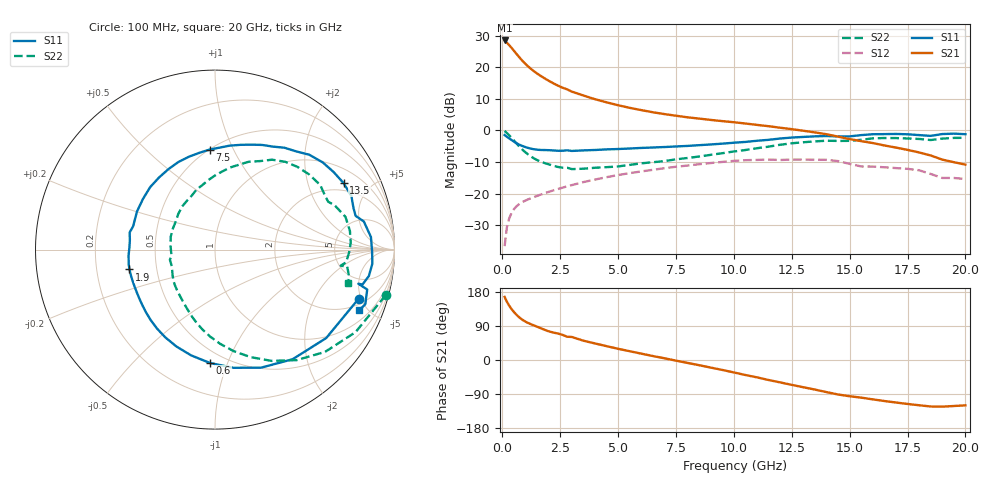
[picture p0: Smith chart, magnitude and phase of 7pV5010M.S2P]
! Infineon Technologies  Discrete & RF Semiconductors
! bfp620
! VCE = 0.50 V,  IC =  10 mA
! Common Emitter S-Parameters:  Sep 2002
# GHz  S  MA  R  50
!  f  S11  S21  S12  S22
! GHz  MAG  ANG  MAG  ANG  MAG  ANG  MAG  ANG
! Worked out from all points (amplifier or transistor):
!   59 points, 100 MHz to 20 GHz, reference 50 ohm
!   highest |S21| = 28.5 dB at 100 MHz (marker M1)
!   |S21| within 3 dB of that: start of sweep to 474.6 MHz
!   unconditionally stable (mu >= 1): 3.938 GHz to 10.17 GHz; 17.11 GHz to end of sweep
!   at 1 GHz: K = 0.51, MSG = 21.6 dB, |S12| = -22.2 dB
!   at 5.5 GHz: K = 1.05, MAG = 8.9 dB, |S12| = -13.5 dB
!   at 20 GHz: K = 1.68, MAG = -2.5 dB, |S12| = -15.4 dB
!   S11 on the Smith chart (normalised r, x): 100 MHz: 2.49, -4.79; 600 MHz: 0.41, -0.87; 1.9 GHz: 0.35, -0.10; 7.5 GHz: 0.50, +0.81; 13.5 GHz: 1.60, +3.40; 20 GHz: 1.58, -4.44
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0.1  0.8462 -18.8  26.47 166.4  0.0148 79.7  0.9837 -15.0
0.2  0.7917 -38.5  24.32 153.5  0.0297 69.7  0.9083 -30.4
0.3  0.7484 -54.7  22.26 143.1  0.0409 63.1  0.8372 -42.9
0.4  0.7062 -68.6  20.22 134.4  0.0497 57.7  0.7652 -53.6
0.5  0.6667 -81.1  18.26 126.8  0.0567 53.2  0.6952 -63.1
0.6  0.6324 -92.5  16.46 120.1  0.0625 49.6  0.6309 -71.7
0.7  0.6042 -102.7  14.86 114.3  0.0672 46.8  0.5744 -79.7
0.8  0.5811 -111.7  13.47 109.2  0.0713 44.6  0.5261 -86.8
1  0.5456 -126.4  11.27 101.2  0.0779 41.8  0.4508 -98.9
1.2  0.5194 -137.8  9.673 95.4  0.0837 40.2  0.3963 -108.6
1.4  0.5017 -147.3  8.47 90.4  0.0893 39.2  0.3563 -117.2
1.9  0.4891 -166.9  6.419 78.0  0.1038 37.1  0.2992 -138.1
2.6  0.4773 173.5  4.75 66.4  0.1245 34.2  0.2575 -160.6
2.8  0.4851 168.7  4.459 61.4  0.1308 33.0  0.2575 -167.4
3.5  0.4837 154.0  3.57 51.0  0.1525 28.7  0.2482 175.9
5  0.5087 127.7  2.504 29.6  0.1973 17.5  0.2696 143.7
7  0.5466 99.0  1.815 4.6  0.2529 0.5  0.3278 113.2
7.5  0.5582 93.1  1.71 -1.7  0.2666 -4.4  0.3493 107.2
10.5  0.6586 60.6  1.287 -39.6  0.3386 -36.3  0.4904 74.4
13.5  0.8065 27.4  0.931 -78.0  0.3444 -70.7  0.6713 38.6
17  0.8803 -5.1  0.536 -112.2  0.2542 -101.8  0.7573 2.9
20  0.8721 -22.7  0.288 -119.7  0.1708 -114.2  0.7637 -14.0
